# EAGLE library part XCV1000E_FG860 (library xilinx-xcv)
xcv1000e_fg860_1532 edit this description Auto generated by make-symbol-device-package-bsdl.ulp Rev. 26 Source: xcv1000e_fg860_1532.bsd
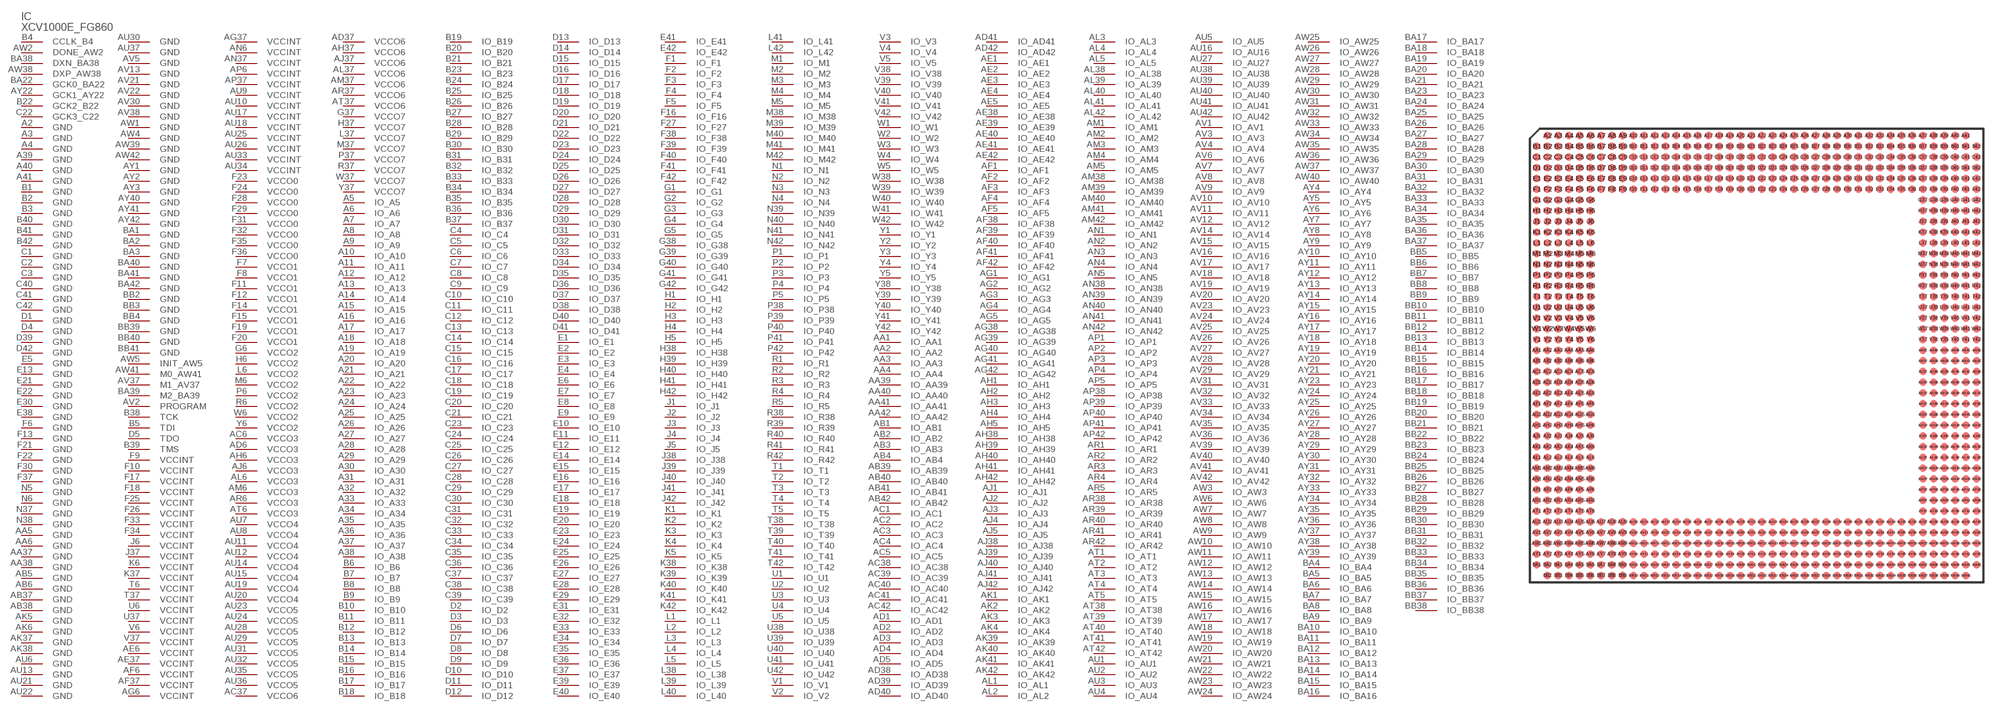
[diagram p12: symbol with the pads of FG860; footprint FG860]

Designator prefix IC

## XCV1000E_FG860 (OC_FARNELL: unknown; OC_NEWARK: unknown)  [FG860]
A2  GND  pwr
A3  GND  pwr
A4  GND  pwr
A5  IO_A5
A6  IO_A6
A7  IO_A7
A8  IO_A8
A9  IO_A9
A10  IO_A10
A11  IO_A11
A12  IO_A12
A13  IO_A13
A14  IO_A14
A15  IO_A15
A16  IO_A16
A17  IO_A17
A18  IO_A18
A19  IO_A19
A20  IO_A20
A21  IO_A21
A22  IO_A22
A23  IO_A23
A24  IO_A24
A25  IO_A25
A26  IO_A26
A27  IO_A27
A28  IO_A28
A29  IO_A29
A30  IO_A30
A31  IO_A31
A32  IO_A32
A33  IO_A33
A34  IO_A34
A35  IO_A35
A36  IO_A36
A37  IO_A37
A38  IO_A38
A39  GND  pwr
A40  GND  pwr
A41  GND  pwr
AA1  IO_AA1
AA2  IO_AA2
AA3  IO_AA3
AA4  IO_AA4
AA5  GND  pwr
AA6  GND  pwr
AA37  GND  pwr
AA38  GND  pwr
AA39  IO_AA39
AA40  IO_AA40
AA41  IO_AA41
AA42  IO_AA42
AB1  IO_AB1
AB2  IO_AB2
AB3  IO_AB3
AB4  IO_AB4
AB5  GND  pwr
AB6  GND  pwr
AB37  GND  pwr
AB38  GND  pwr
AB39  IO_AB39
AB40  IO_AB40
AB41  IO_AB41
AB42  IO_AB42
AC1  IO_AC1
AC2  IO_AC2
AC3  IO_AC3
AC4  IO_AC4
AC5  IO_AC5
AC6  VCCO3  pwr
AC37  VCCO6  pwr
AC38  IO_AC38
AC39  IO_AC39
AC40  IO_AC40
AC41  IO_AC41
AC42  IO_AC42
AD1  IO_AD1
AD2  IO_AD2
AD3  IO_AD3
AD4  IO_AD4
AD5  IO_AD5
AD6  VCCO3  pwr
AD37  VCCO6  pwr
AD38  IO_AD38
AD39  IO_AD39
AD40  IO_AD40
AD41  IO_AD41
AD42  IO_AD42
AE1  IO_AE1
AE2  IO_AE2
AE3  IO_AE3
AE4  IO_AE4
AE5  IO_AE5
AE6  VCCINT  pwr
AE37  VCCINT  pwr
AE38  IO_AE38
AE39  IO_AE39
AE40  IO_AE40
AE41  IO_AE41
AE42  IO_AE42
AF1  IO_AF1
AF2  IO_AF2
AF3  IO_AF3
AF4  IO_AF4
AF5  IO_AF5
AF6  VCCINT  pwr
AF37  VCCINT  pwr
AF38  IO_AF38
AF39  IO_AF39
AF40  IO_AF40
AF41  IO_AF41
AF42  IO_AF42
AG1  IO_AG1
AG2  IO_AG2
AG3  IO_AG3
AG4  IO_AG4
AG5  IO_AG5
AG6  VCCINT  pwr
AG37  VCCINT  pwr
AG38  IO_AG38
AG39  IO_AG39
AG40  IO_AG40
AG41  IO_AG41
AG42  IO_AG42
AH1  IO_AH1
AH2  IO_AH2
AH3  IO_AH3
AH4  IO_AH4
AH5  IO_AH5
AH6  VCCO3  pwr
AH37  VCCO6  pwr
AH38  IO_AH38
AH39  IO_AH39
AH40  IO_AH40
AH41  IO_AH41
AH42  IO_AH42
AJ1  IO_AJ1
AJ2  IO_AJ2
AJ3  IO_AJ3
AJ4  IO_AJ4
AJ5  IO_AJ5
AJ6  VCCO3  pwr
AJ37  VCCO6  pwr
AJ38  IO_AJ38
AJ39  IO_AJ39
AJ40  IO_AJ40
AJ41  IO_AJ41
AJ42  IO_AJ42
AK1  IO_AK1
AK2  IO_AK2
AK3  IO_AK3
AK4  IO_AK4
AK5  GND  pwr
AK6  GND  pwr
AK37  GND  pwr
AK38  GND  pwr
AK39  IO_AK39
AK40  IO_AK40
AK41  IO_AK41
AK42  IO_AK42
AL1  IO_AL1
AL2  IO_AL2
AL3  IO_AL3
AL4  IO_AL4
AL5  IO_AL5
AL6  VCCO3  pwr
AL37  VCCO6  pwr
AL38  IO_AL38
AL39  IO_AL39
AL40  IO_AL40
AL41  IO_AL41
AL42  IO_AL42
AM1  IO_AM1
AM2  IO_AM2
AM3  IO_AM3
AM4  IO_AM4
AM5  IO_AM5
AM6  VCCO3  pwr
AM37  VCCO6  pwr
AM38  IO_AM38
AM39  IO_AM39
AM40  IO_AM40
AM41  IO_AM41
AM42  IO_AM42
AN1  IO_AN1
AN2  IO_AN2
AN3  IO_AN3
AN4  IO_AN4
AN5  IO_AN5
AN6  VCCINT  pwr
AN37  VCCINT  pwr
AN38  IO_AN38
AN39  IO_AN39
AN40  IO_AN40
AN41  IO_AN41
AN42  IO_AN42
AP1  IO_AP1
AP2  IO_AP2
AP3  IO_AP3
AP4  IO_AP4
AP5  IO_AP5
AP6  VCCINT  pwr
AP37  VCCINT  pwr
AP38  IO_AP38
AP39  IO_AP39
AP40  IO_AP40
AP41  IO_AP41
AP42  IO_AP42
AR1  IO_AR1
AR2  IO_AR2
AR3  IO_AR3
AR4  IO_AR4
AR5  IO_AR5
AR6  VCCO3  pwr
AR37  VCCO6  pwr
AR38  IO_AR38
AR39  IO_AR39
AR40  IO_AR40
AR41  IO_AR41
AR42  IO_AR42
AT1  IO_AT1
AT2  IO_AT2
AT3  IO_AT3
AT4  IO_AT4
AT5  IO_AT5
AT6  VCCO3  pwr
AT37  VCCO6  pwr
AT38  IO_AT38
AT39  IO_AT39
AT40  IO_AT40
AT41  IO_AT41
AT42  IO_AT42
AU1  IO_AU1
AU2  IO_AU2
AU3  IO_AU3
AU4  IO_AU4
AU5  IO_AU5
AU6  GND  pwr
AU7  VCCO4  pwr
AU8  VCCO4  pwr
AU9  VCCINT  pwr
AU10  VCCINT  pwr
AU11  VCCO4  pwr
AU12  VCCO4  pwr
AU13  GND  pwr
AU14  VCCO4  pwr
AU15  VCCO4  pwr
AU16  IO_AU16
AU17  VCCINT  pwr
AU18  VCCINT  pwr
AU19  VCCO4  pwr
AU20  VCCO4  pwr
AU21  GND  pwr
AU22  GND  pwr
AU23  VCCO5  pwr
AU24  VCCO5  pwr
AU25  VCCINT  pwr
AU26  VCCINT  pwr
AU27  IO_AU27
AU28  VCCO5  pwr
AU29  VCCO5  pwr
AU30  GND  pwr
AU31  VCCO5  pwr
AU32  VCCO5  pwr
AU33  VCCINT  pwr
AU34  VCCINT  pwr
AU35  VCCO5  pwr
AU36  VCCO5  pwr
AU37  GND  pwr
AU38  IO_AU38
AU39  IO_AU39
AU40  IO_AU40
AU41  IO_AU41
AU42  IO_AU42
AV1  IO_AV1
AV2  PROGRAM  in
AV3  IO_AV3
AV4  IO_AV4
AV5  GND  pwr
AV6  IO_AV6
AV7  IO_AV7
AV8  IO_AV8
AV9  IO_AV9
AV10  IO_AV10
AV11  IO_AV11
AV12  IO_AV12
AV13  GND  pwr
AV14  IO_AV14
AV15  IO_AV15
AV16  IO_AV16
AV17  IO_AV17
AV18  IO_AV18
AV19  IO_AV19
AV20  IO_AV20
AV21  GND  pwr
AV22  GND  pwr
AV23  IO_AV23
AV24  IO_AV24
AV25  IO_AV25
AV26  IO_AV26
AV27  IO_AV27
AV28  IO_AV28
AV29  IO_AV29
AV30  GND  pwr
AV31  IO_AV31
AV32  IO_AV32
AV33  IO_AV33
AV34  IO_AV34
AV35  IO_AV35
AV36  IO_AV36
AV37  M1_AV37  in
AV38  GND  pwr
AV39  IO_AV39
AV40  IO_AV40
AV41  IO_AV41
AV42  IO_AV42
AW1  GND  pwr
AW2  DONE_AW2
AW3  IO_AW3
AW4  GND  pwr
AW5  INIT_AW5
AW6  IO_AW6
AW7  IO_AW7
AW8  IO_AW8
AW9  IO_AW9
AW10  IO_AW10
AW11  IO_AW11
AW12  IO_AW12
AW13  IO_AW13
AW14  IO_AW14
AW15  IO_AW15
AW16  IO_AW16
AW17  IO_AW17
AW18  IO_AW18
AW19  IO_AW19
AW20  IO_AW20
AW21  IO_AW21
AW22  IO_AW22
AW23  IO_AW23
AW24  IO_AW24
AW25  IO_AW25
AW26  IO_AW26
AW27  IO_AW27
AW28  IO_AW28
AW29  IO_AW29
AW30  IO_AW30
AW31  IO_AW31
AW32  IO_AW32
AW33  IO_AW33
AW34  IO_AW34
AW35  IO_AW35
AW36  IO_AW36
AW37  IO_AW37
AW38  DXP_AW38  pas
AW39  GND  pwr
AW40  IO_AW40
AW41  M0_AW41  in
AW42  GND  pwr
AY1  GND  pwr
AY2  GND  pwr
AY3  GND  pwr
AY4  IO_AY4
AY5  IO_AY5
AY6  IO_AY6
AY7  IO_AY7
AY8  IO_AY8
AY9  IO_AY9
AY10  IO_AY10
AY11  IO_AY11
AY12  IO_AY12
AY13  IO_AY13
AY14  IO_AY14
AY15  IO_AY15
AY16  IO_AY16
AY17  IO_AY17
AY18  IO_AY18
AY19  IO_AY19
AY20  IO_AY20
AY21  IO_AY21
AY22  GCK1_AY22  in
AY23  IO_AY23
AY24  IO_AY24
AY25  IO_AY25
AY26  IO_AY26
AY27  IO_AY27
AY28  IO_AY28
AY29  IO_AY29
AY30  IO_AY30
AY31  IO_AY31
AY32  IO_AY32
AY33  IO_AY33
AY34  IO_AY34
AY35  IO_AY35
AY36  IO_AY36
AY37  IO_AY37
AY38  IO_AY38
AY39  IO_AY39
AY40  GND  pwr
AY41  GND  pwr
AY42  GND  pwr
B1  GND  pwr
B2  GND  pwr
B3  GND  pwr
B4  CCLK_B4
B5  TDI  in
B6  IO_B6
B7  IO_B7
B8  IO_B8
B9  IO_B9
B10  IO_B10
B11  IO_B11
B12  IO_B12
B13  IO_B13
B14  IO_B14
B15  IO_B15
B16  IO_B16
B17  IO_B17
B18  IO_B18
B19  IO_B19
B20  IO_B20
B21  IO_B21
B22  GCK2_B22  in
B23  IO_B23
B24  IO_B24
B25  IO_B25
B26  IO_B26
B27  IO_B27
B28  IO_B28
B29  IO_B29
B30  IO_B30
B31  IO_B31
B32  IO_B32
B33  IO_B33
B34  IO_B34
B35  IO_B35
B36  IO_B36
B37  IO_B37
B38  TCK  in
B39  TMS  in
B40  GND  pwr
B41  GND  pwr
B42  GND  pwr
BA1  GND  pwr
BA2  GND  pwr
BA3  GND  pwr
BA4  IO_BA4
BA5  IO_BA5
BA6  IO_BA6
BA7  IO_BA7
BA8  IO_BA8
BA9  IO_BA9
BA10  IO_BA10
BA11  IO_BA11
BA12  IO_BA12
BA13  IO_BA13
BA14  IO_BA14
BA15  IO_BA15
BA16  IO_BA16
BA17  IO_BA17
BA18  IO_BA18
BA19  IO_BA19
BA20  IO_BA20
BA21  IO_BA21
BA22  GCK0_BA22  in
BA23  IO_BA23
BA24  IO_BA24
BA25  IO_BA25
BA26  IO_BA26
BA27  IO_BA27
BA28  IO_BA28
BA29  IO_BA29
BA30  IO_BA30
BA31  IO_BA31
BA32  IO_BA32
BA33  IO_BA33
BA34  IO_BA34
BA35  IO_BA35
BA36  IO_BA36
BA37  IO_BA37
BA38  DXN_BA38  pas
BA39  M2_BA39  in
BA40  GND  pwr
BA41  GND  pwr
BA42  GND  pwr
BB2  GND  pwr
BB3  GND  pwr
BB4  GND  pwr
BB5  IO_BB5
BB6  IO_BB6
BB7  IO_BB7
BB8  IO_BB8
BB9  IO_BB9
BB10  IO_BB10
BB11  IO_BB11
BB12  IO_BB12
BB13  IO_BB13
BB14  IO_BB14
BB15  IO_BB15
BB16  IO_BB16
BB17  IO_BB17
BB18  IO_BB18
BB19  IO_BB19
BB20  IO_BB20
BB21  IO_BB21
BB22  IO_BB22
BB23  IO_BB23
BB24  IO_BB24
BB25  IO_BB25
BB26  IO_BB26
BB27  IO_BB27
BB28  IO_BB28
BB29  IO_BB29
BB30  IO_BB30
BB31  IO_BB31
BB32  IO_BB32
BB33  IO_BB33
BB34  IO_BB34
BB35  IO_BB35
BB36  IO_BB36
BB37  IO_BB37
BB38  IO_BB38
BB39  GND  pwr
BB40  GND  pwr
BB41  GND  pwr
C1  GND  pwr
C2  GND  pwr
C3  GND  pwr
C4  IO_C4
C5  IO_C5
C6  IO_C6
C7  IO_C7
C8  IO_C8
C9  IO_C9
C10  IO_C10
C11  IO_C11
C12  IO_C12
C13  IO_C13
C14  IO_C14
C15  IO_C15
C16  IO_C16
C17  IO_C17
C18  IO_C18
C19  IO_C19
C20  IO_C20
C21  IO_C21
C22  GCK3_C22  in
C23  IO_C23
C24  IO_C24
C25  IO_C25
C26  IO_C26
C27  IO_C27
C28  IO_C28
C29  IO_C29
C30  IO_C30
C31  IO_C31
C32  IO_C32
C33  IO_C33
C34  IO_C34
C35  IO_C35
C36  IO_C36
C37  IO_C37
C38  IO_C38
C39  IO_C39
C40  GND  pwr
C41  GND  pwr
C42  GND  pwr
D1  GND  pwr
D2  IO_D2
D3  IO_D3
D4  GND  pwr
D5  TDO  out
D6  IO_D6
D7  IO_D7
D8  IO_D8
D9  IO_D9
D10  IO_D10
D11  IO_D11
D12  IO_D12
D13  IO_D13
D14  IO_D14
D15  IO_D15
D16  IO_D16
D17  IO_D17
D18  IO_D18
D19  IO_D19
D20  IO_D20
D21  IO_D21
D22  IO_D22
D23  IO_D23
D24  IO_D24
D25  IO_D25
D26  IO_D26
D27  IO_D27
D28  IO_D28
D29  IO_D29
D30  IO_D30
D31  IO_D31
D32  IO_D32
D33  IO_D33
D34  IO_D34
D35  IO_D35
D36  IO_D36
D37  IO_D37
D38  IO_D38
D39  GND  pwr
D40  IO_D40
D41  IO_D41
D42  GND  pwr
E1  IO_E1
E2  IO_E2
E3  IO_E3
E4  IO_E4
E5  GND  pwr
E6  IO_E6
E7  IO_E7
E8  IO_E8
E9  IO_E9
E10  IO_E10
E11  IO_E11
E12  IO_E12
E13  GND  pwr
E14  IO_E14
E15  IO_E15
E16  IO_E16
E17  IO_E17
E18  IO_E18
E19  IO_E19
E20  IO_E20
E21  GND  pwr
E22  GND  pwr
E23  IO_E23
E24  IO_E24
E25  IO_E25
E26  IO_E26
E27  IO_E27
E28  IO_E28
E29  IO_E29
E30  GND  pwr
E31  IO_E31
E32  IO_E32
E33  IO_E33
E34  IO_E34
E35  IO_E35
E36  IO_E36
E37  IO_E37
E38  GND  pwr
E39  IO_E39
E40  IO_E40
E41  IO_E41
E42  IO_E42
F1  IO_F1
F2  IO_F2
F3  IO_F3
F4  IO_F4
F5  IO_F5
F6  GND  pwr
F7  VCCO1  pwr
F8  VCCO1  pwr
F9  VCCINT  pwr
F10  VCCINT  pwr
F11  VCCO1  pwr
F12  VCCO1  pwr
F13  GND  pwr
F14  VCCO1  pwr
F15  VCCO1  pwr
F16  IO_F16
F17  VCCINT  pwr
F18  VCCINT  pwr
F19  VCCO1  pwr
F20  VCCO1  pwr
F21  GND  pwr
F22  GND  pwr
F23  VCCO0  pwr
F24  VCCO0  pwr
F25  VCCINT  pwr
F26  VCCINT  pwr
F27  IO_F27
F28  VCCO0  pwr
F29  VCCO0  pwr
F30  GND  pwr
F31  VCCO0  pwr
F32  VCCO0  pwr
F33  VCCINT  pwr
F34  VCCINT  pwr
F35  VCCO0  pwr
F36  VCCO0  pwr
F37  GND  pwr
F38  IO_F38
F39  IO_F39
F40  IO_F40
F41  IO_F41
F42  IO_F42
G1  IO_G1
G2  IO_G2
G3  IO_G3
G4  IO_G4
G5  IO_G5
G6  VCCO2  pwr
G37  VCCO7  pwr
G38  IO_G38
G39  IO_G39
G40  IO_G40
G41  IO_G41
G42  IO_G42
H1  IO_H1
H2  IO_H2
H3  IO_H3
H4  IO_H4
H5  IO_H5
H6  VCCO2  pwr
H37  VCCO7  pwr
H38  IO_H38
H39  IO_H39
H40  IO_H40
H41  IO_H41
H42  IO_H42
J1  IO_J1
J2  IO_J2
J3  IO_J3
J4  IO_J4
J5  IO_J5
J6  VCCINT  pwr
J37  VCCINT  pwr
J38  IO_J38
J39  IO_J39
J40  IO_J40
J41  IO_J41
J42  IO_J42
K1  IO_K1
K2  IO_K2
K3  IO_K3
K4  IO_K4
K5  IO_K5
K6  VCCINT  pwr
K37  VCCINT  pwr
K38  IO_K38
K39  IO_K39
K40  IO_K40
K41  IO_K41
K42  IO_K42
L1  IO_L1
L2  IO_L2
L3  IO_L3
L4  IO_L4
L5  IO_L5
L6  VCCO2  pwr
L37  VCCO7  pwr
L38  IO_L38
L39  IO_L39
L40  IO_L40
L41  IO_L41
L42  IO_L42
M1  IO_M1
M2  IO_M2
M3  IO_M3
M4  IO_M4
M5  IO_M5
M6  VCCO2  pwr
M37  VCCO7  pwr
M38  IO_M38
M39  IO_M39
M40  IO_M40
M41  IO_M41
M42  IO_M42
N1  IO_N1
N2  IO_N2
N3  IO_N3
N4  IO_N4
N5  GND  pwr
N6  GND  pwr
N37  GND  pwr
N38  GND  pwr
N39  IO_N39
N40  IO_N40
N41  IO_N41
N42  IO_N42
P1  IO_P1
P2  IO_P2
P3  IO_P3
P4  IO_P4
P5  IO_P5
P6  VCCO2  pwr
P37  VCCO7  pwr
P38  IO_P38
P39  IO_P39
P40  IO_P40
P41  IO_P41
P42  IO_P42
R1  IO_R1
R2  IO_R2
R3  IO_R3
R4  IO_R4
R5  IO_R5
R6  VCCO2  pwr
R37  VCCO7  pwr
R38  IO_R38
R39  IO_R39
R40  IO_R40
R41  IO_R41
R42  IO_R42
T1  IO_T1
T2  IO_T2
T3  IO_T3
T4  IO_T4
T5  IO_T5
T6  VCCINT  pwr
T37  VCCINT  pwr
T38  IO_T38
T39  IO_T39
T40  IO_T40
T41  IO_T41
T42  IO_T42
U1  IO_U1
U2  IO_U2
U3  IO_U3
U4  IO_U4
U5  IO_U5
U6  VCCINT  pwr
U37  VCCINT  pwr
U38  IO_U38
U39  IO_U39
U40  IO_U40
U41  IO_U41
U42  IO_U42
V1  IO_V1
V2  IO_V2
V3  IO_V3
V4  IO_V4
V5  IO_V5
V6  VCCINT  pwr
V37  VCCINT  pwr
V38  IO_V38
V39  IO_V39
V40  IO_V40
V41  IO_V41
V42  IO_V42
W1  IO_W1
W2  IO_W2
W3  IO_W3
W4  IO_W4
W5  IO_W5
W6  VCCO2  pwr
W37  VCCO7  pwr
W38  IO_W38
W39  IO_W39
W40  IO_W40
W41  IO_W41
W42  IO_W42
Y1  IO_Y1
Y2  IO_Y2
Y3  IO_Y3
Y4  IO_Y4
Y5  IO_Y5
Y6  VCCO2  pwr
Y37  VCCO7  pwr
Y38  IO_Y38
Y39  IO_Y39
Y40  IO_Y40
Y41  IO_Y41
Y42  IO_Y42

## Footprint FG860 (pad centres in mm)
xcv1000e_fg860_1532 edit this description Auto generated by make-symbol-device-package-bsdl.ulp Rev. 26 Source: xcv1000e_fg860_1532.bsd
smd 0.7 x 0.7: A2 -19.5,20.5; A3 -18.5,20.5; A4 -17.5,20.5; A5 -16.5,20.5; A6 -15.5,20.5; A7 -14.5,20.5; A8 -13.5,20.5; A9 -12.5,20.5; A10 -11.5,20.5; A11 -10.5,20.5; A12 -9.5,20.5; A13 -8.5,20.5; A14 -7.5,20.5; A15 -6.5,20.5; A16 -5.5,20.5; A17 -4.5,20.5; A18 -3.5,20.5; A19 -2.5,20.5; A20 -1.5,20.5; A21 -0.5,20.5; A22 0.5,20.5; A23 1.5,20.5; A24 2.5,20.5; A25 3.5,20.5; A26 4.5,20.5; A27 5.5,20.5; A28 6.5,20.5; A29 7.5,20.5; A30 8.5,20.5; A31 9.5,20.5; A32 10.5,20.5; A33 11.5,20.5; A34 12.5,20.5; A35 13.5,20.5; A36 14.5,20.5; A37 15.5,20.5; A38 16.5,20.5; A39 17.5,20.5; A40 18.5,20.5; A41 19.5,20.5; AA1 -20.5,0.5; AA2 -19.5,0.5; AA3 -18.5,0.5; AA4 -17.5,0.5; AA5 -16.5,0.5; AA6 -15.5,0.5; AA37 15.5,0.5; AA38 16.5,0.5; AA39 17.5,0.5; AA40 18.5,0.5; AA41 19.5,0.5; AA42 20.5,0.5; AB1 -20.5,-0.5; AB2 -19.5,-0.5; AB3 -18.5,-0.5; AB4 -17.5,-0.5; AB5 -16.5,-0.5; AB6 -15.5,-0.5; AB37 15.5,-0.5; AB38 16.5,-0.5; AB39 17.5,-0.5; AB40 18.5,-0.5; AB41 19.5,-0.5; AB42 20.5,-0.5; AC1 -20.5,-1.5; AC2 -19.5,-1.5; AC3 -18.5,-1.5; AC4 -17.5,-1.5; AC5 -16.5,-1.5; AC6 -15.5,-1.5; AC37 15.5,-1.5; AC38 16.5,-1.5; AC39 17.5,-1.5; AC40 18.5,-1.5; AC41 19.5,-1.5; AC42 20.5,-1.5; AD1 -20.5,-2.5; AD2 -19.5,-2.5; AD3 -18.5,-2.5; AD4 -17.5,-2.5; AD5 -16.5,-2.5; AD6 -15.5,-2.5; AD37 15.5,-2.5; AD38 16.5,-2.5; AD39 17.5,-2.5; AD40 18.5,-2.5; AD41 19.5,-2.5; AD42 20.5,-2.5; AE1 -20.5,-3.5; AE2 -19.5,-3.5; AE3 -18.5,-3.5; AE4 -17.5,-3.5; AE5 -16.5,-3.5; AE6 -15.5,-3.5; AE37 15.5,-3.5; AE38 16.5,-3.5; AE39 17.5,-3.5; AE40 18.5,-3.5; AE41 19.5,-3.5; AE42 20.5,-3.5; AF1 -20.5,-4.5; AF2 -19.5,-4.5; AF3 -18.5,-4.5; AF4 -17.5,-4.5; AF5 -16.5,-4.5; AF6 -15.5,-4.5; AF37 15.5,-4.5; AF38 16.5,-4.5; AF39 17.5,-4.5; AF40 18.5,-4.5; AF41 19.5,-4.5; AF42 20.5,-4.5; AG1 -20.5,-5.5; AG2 -19.5,-5.5; AG3 -18.5,-5.5; AG4 -17.5,-5.5; AG5 -16.5,-5.5; AG6 -15.5,-5.5; AG37 15.5,-5.5; AG38 16.5,-5.5; AG39 17.5,-5.5; AG40 18.5,-5.5; AG41 19.5,-5.5; AG42 20.5,-5.5; AH1 -20.5,-6.5; AH2 -19.5,-6.5; AH3 -18.5,-6.5; AH4 -17.5,-6.5; AH5 -16.5,-6.5; AH6 -15.5,-6.5; AH37 15.5,-6.5; AH38 16.5,-6.5; AH39 17.5,-6.5; AH40 18.5,-6.5; AH41 19.5,-6.5; AH42 20.5,-6.5; AJ1 -20.5,-7.5; AJ2 -19.5,-7.5; AJ3 -18.5,-7.5; AJ4 -17.5,-7.5; AJ5 -16.5,-7.5; AJ6 -15.5,-7.5; AJ37 15.5,-7.5; AJ38 16.5,-7.5; AJ39 17.5,-7.5; AJ40 18.5,-7.5; AJ41 19.5,-7.5; AJ42 20.5,-7.5; AK1 -20.5,-8.5; AK2 -19.5,-8.5; AK3 -18.5,-8.5; AK4 -17.5,-8.5; AK5 -16.5,-8.5; AK6 -15.5,-8.5; AK37 15.5,-8.5; AK38 16.5,-8.5; AK39 17.5,-8.5; AK40 18.5,-8.5; AK41 19.5,-8.5; AK42 20.5,-8.5; AL1 -20.5,-9.5; AL2 -19.5,-9.5; AL3 -18.5,-9.5; AL4 -17.5,-9.5; AL5 -16.5,-9.5; AL6 -15.5,-9.5; AL37 15.5,-9.5; AL38 16.5,-9.5; AL39 17.5,-9.5; AL40 18.5,-9.5; AL41 19.5,-9.5; AL42 20.5,-9.5; AM1 -20.5,-10.5; AM2 -19.5,-10.5; AM3 -18.5,-10.5; AM4 -17.5,-10.5; AM5 -16.5,-10.5; AM6 -15.5,-10.5; AM37 15.5,-10.5; AM38 16.5,-10.5; AM39 17.5,-10.5; AM40 18.5,-10.5; AM41 19.5,-10.5; AM42 20.5,-10.5; AN1 -20.5,-11.5; AN2 -19.5,-11.5; AN3 -18.5,-11.5; AN4 -17.5,-11.5; AN5 -16.5,-11.5; AN6 -15.5,-11.5; AN37 15.5,-11.5; AN38 16.5,-11.5; AN39 17.5,-11.5; AN40 18.5,-11.5; AN41 19.5,-11.5; AN42 20.5,-11.5; AP1 -20.5,-12.5; AP2 -19.5,-12.5; AP3 -18.5,-12.5; AP4 -17.5,-12.5; AP5 -16.5,-12.5; AP6 -15.5,-12.5; AP37 15.5,-12.5; AP38 16.5,-12.5; AP39 17.5,-12.5; AP40 18.5,-12.5; AP41 19.5,-12.5; AP42 20.5,-12.5; AR1 -20.5,-13.5; AR2 -19.5,-13.5; AR3 -18.5,-13.5; AR4 -17.5,-13.5; AR5 -16.5,-13.5; AR6 -15.5,-13.5; AR37 15.5,-13.5; AR38 16.5,-13.5; AR39 17.5,-13.5; AR40 18.5,-13.5; AR41 19.5,-13.5; AR42 20.5,-13.5; AT1 -20.5,-14.5; AT2 -19.5,-14.5; AT3 -18.5,-14.5; AT4 -17.5,-14.5; AT5 -16.5,-14.5; AT6 -15.5,-14.5; AT37 15.5,-14.5; AT38 16.5,-14.5; AT39 17.5,-14.5; AT40 18.5,-14.5; AT41 19.5,-14.5; AT42 20.5,-14.5; AU1 -20.5,-15.5; AU2 -19.5,-15.5; AU3 -18.5,-15.5; AU4 -17.5,-15.5; AU5 -16.5,-15.5; AU6 -15.5,-15.5; AU7 -14.5,-15.5; AU8 -13.5,-15.5; AU9 -12.5,-15.5; AU10 -11.5,-15.5; AU11 -10.5,-15.5; AU12 -9.5,-15.5; AU13 -8.5,-15.5; AU14 -7.5,-15.5; AU15 -6.5,-15.5; AU16 -5.5,-15.5; AU17 -4.5,-15.5; AU18 -3.5,-15.5; AU19 -2.5,-15.5; AU20 -1.5,-15.5; AU21 -0.5,-15.5; AU22 0.5,-15.5; AU23 1.5,-15.5; AU24 2.5,-15.5; AU25 3.5,-15.5; AU26 4.5,-15.5; AU27 5.5,-15.5; AU28 6.5,-15.5; AU29 7.5,-15.5; AU30 8.5,-15.5; AU31 9.5,-15.5; AU32 10.5,-15.5; AU33 11.5,-15.5; AU34 12.5,-15.5; AU35 13.5,-15.5; AU36 14.5,-15.5; AU37 15.5,-15.5; AU38 16.5,-15.5; AU39 17.5,-15.5; AU40 18.5,-15.5; AU41 19.5,-15.5; AU42 20.5,-15.5; AV1 -20.5,-16.5; AV2 -19.5,-16.5; AV3 -18.5,-16.5; AV4 -17.5,-16.5; AV5 -16.5,-16.5; AV6 -15.5,-16.5; AV7 -14.5,-16.5; AV8 -13.5,-16.5; AV9 -12.5,-16.5; AV10 -11.5,-16.5; AV11 -10.5,-16.5; AV12 -9.5,-16.5; AV13 -8.5,-16.5; AV14 -7.5,-16.5; AV15 -6.5,-16.5; AV16 -5.5,-16.5; AV17 -4.5,-16.5; AV18 -3.5,-16.5; AV19 -2.5,-16.5; AV20 -1.5,-16.5; AV21 -0.5,-16.5; AV22 0.5,-16.5; AV23 1.5,-16.5; AV24 2.5,-16.5; AV25 3.5,-16.5; AV26 4.5,-16.5; AV27 5.5,-16.5; AV28 6.5,-16.5; AV29 7.5,-16.5; AV30 8.5,-16.5; AV31 9.5,-16.5; AV32 10.5,-16.5; AV33 11.5,-16.5; AV34 12.5,-16.5; AV35 13.5,-16.5; AV36 14.5,-16.5; AV37 15.5,-16.5; AV38 16.5,-16.5; AV39 17.5,-16.5; AV40 18.5,-16.5; AV41 19.5,-16.5; AV42 20.5,-16.5; AW1 -20.5,-17.5; AW2 -19.5,-17.5; AW3 -18.5,-17.5; AW4 -17.5,-17.5; AW5 -16.5,-17.5; AW6 -15.5,-17.5; AW7 -14.5,-17.5; AW8 -13.5,-17.5; AW9 -12.5,-17.5; AW10 -11.5,-17.5; AW11 -10.5,-17.5; AW12 -9.5,-17.5; AW13 -8.5,-17.5; AW14 -7.5,-17.5; AW15 -6.5,-17.5; AW16 -5.5,-17.5; AW17 -4.5,-17.5; AW18 -3.5,-17.5; AW19 -2.5,-17.5; AW20 -1.5,-17.5; AW21 -0.5,-17.5; AW22 0.5,-17.5; AW23 1.5,-17.5; AW24 2.5,-17.5; AW25 3.5,-17.5; AW26 4.5,-17.5; AW27 5.5,-17.5; AW28 6.5,-17.5; AW29 7.5,-17.5; AW30 8.5,-17.5; AW31 9.5,-17.5; AW32 10.5,-17.5; AW33 11.5,-17.5; AW34 12.5,-17.5; AW35 13.5,-17.5; AW36 14.5,-17.5; AW37 15.5,-17.5; AW38 16.5,-17.5; AW39 17.5,-17.5; AW40 18.5,-17.5; AW41 19.5,-17.5; AW42 20.5,-17.5; AY1 -20.5,-18.5; AY2 -19.5,-18.5; AY3 -18.5,-18.5; AY4 -17.5,-18.5; AY5 -16.5,-18.5; AY6 -15.5,-18.5; AY7 -14.5,-18.5; AY8 -13.5,-18.5; AY9 -12.5,-18.5; AY10 -11.5,-18.5; AY11 -10.5,-18.5; AY12 -9.5,-18.5; AY13 -8.5,-18.5; AY14 -7.5,-18.5; AY15 -6.5,-18.5; AY16 -5.5,-18.5; AY17 -4.5,-18.5; AY18 -3.5,-18.5; AY19 -2.5,-18.5; AY20 -1.5,-18.5; AY21 -0.5,-18.5; AY22 0.5,-18.5; AY23 1.5,-18.5; AY24 2.5,-18.5; AY25 3.5,-18.5; AY26 4.5,-18.5; AY27 5.5,-18.5; AY28 6.5,-18.5; AY29 7.5,-18.5; AY30 8.5,-18.5; AY31 9.5,-18.5; AY32 10.5,-18.5; AY33 11.5,-18.5; AY34 12.5,-18.5; AY35 13.5,-18.5; AY36 14.5,-18.5; AY37 15.5,-18.5; AY38 16.5,-18.5; AY39 17.5,-18.5; AY40 18.5,-18.5; AY41 19.5,-18.5; AY42 20.5,-18.5; B1 -20.5,19.5; B2 -19.5,19.5; B3 -18.5,19.5; B4 -17.5,19.5; B5 -16.5,19.5; B6 -15.5,19.5; B7 -14.5,19.5; B8 -13.5,19.5; B9 -12.5,19.5; B10 -11.5,19.5; B11 -10.5,19.5; B12 -9.5,19.5; B13 -8.5,19.5; B14 -7.5,19.5; B15 -6.5,19.5; B16 -5.5,19.5; B17 -4.5,19.5; B18 -3.5,19.5; B19 -2.5,19.5; B20 -1.5,19.5; B21 -0.5,19.5; B22 0.5,19.5; B23 1.5,19.5; B24 2.5,19.5; B25 3.5,19.5; B26 4.5,19.5; B27 5.5,19.5; B28 6.5,19.5; B29 7.5,19.5; B30 8.5,19.5; B31 9.5,19.5; B32 10.5,19.5; B33 11.5,19.5; B34 12.5,19.5; B35 13.5,19.5; B36 14.5,19.5; B37 15.5,19.5; B38 16.5,19.5; B39 17.5,19.5; B40 18.5,19.5; B41 19.5,19.5; B42 20.5,19.5; BA1 -20.5,-19.5; BA2 -19.5,-19.5; BA3 -18.5,-19.5; BA4 -17.5,-19.5; BA5 -16.5,-19.5; BA6 -15.5,-19.5; BA7 -14.5,-19.5; BA8 -13.5,-19.5; BA9 -12.5,-19.5; BA10 -11.5,-19.5; BA11 -10.5,-19.5; BA12 -9.5,-19.5; BA13 -8.5,-19.5; BA14 -7.5,-19.5; BA15 -6.5,-19.5; BA16 -5.5,-19.5; BA17 -4.5,-19.5; BA18 -3.5,-19.5; BA19 -2.5,-19.5; BA20 -1.5,-19.5; BA21 -0.5,-19.5; BA22 0.5,-19.5; BA23 1.5,-19.5; BA24 2.5,-19.5; BA25 3.5,-19.5; BA26 4.5,-19.5; BA27 5.5,-19.5; BA28 6.5,-19.5; BA29 7.5,-19.5; BA30 8.5,-19.5; BA31 9.5,-19.5; BA32 10.5,-19.5; BA33 11.5,-19.5; BA34 12.5,-19.5; BA35 13.5,-19.5; BA36 14.5,-19.5; BA37 15.5,-19.5; BA38 16.5,-19.5; BA39 17.5,-19.5; BA40 18.5,-19.5; BA41 19.5,-19.5; BA42 20.5,-19.5; BB2 -19.5,-20.5; BB3 -18.5,-20.5; BB4 -17.5,-20.5; BB5 -16.5,-20.5; BB6 -15.5,-20.5; BB7 -14.5,-20.5; BB8 -13.5,-20.5; BB9 -12.5,-20.5; BB10 -11.5,-20.5; BB11 -10.5,-20.5; BB12 -9.5,-20.5; BB13 -8.5,-20.5; BB14 -7.5,-20.5; BB15 -6.5,-20.5; BB16 -5.5,-20.5; BB17 -4.5,-20.5; BB18 -3.5,-20.5; BB19 -2.5,-20.5; BB20 -1.5,-20.5; BB21 -0.5,-20.5; BB22 0.5,-20.5; BB23 1.5,-20.5; BB24 2.5,-20.5; BB25 3.5,-20.5; BB26 4.5,-20.5; BB27 5.5,-20.5; BB28 6.5,-20.5; BB29 7.5,-20.5; BB30 8.5,-20.5; BB31 9.5,-20.5; BB32 10.5,-20.5; BB33 11.5,-20.5; BB34 12.5,-20.5; BB35 13.5,-20.5; BB36 14.5,-20.5; BB37 15.5,-20.5; BB38 16.5,-20.5; BB39 17.5,-20.5; BB40 18.5,-20.5; BB41 19.5,-20.5; C1 -20.5,18.5; C2 -19.5,18.5; C3 -18.5,18.5; C4 -17.5,18.5; C5 -16.5,18.5; C6 -15.5,18.5; C7 -14.5,18.5; C8 -13.5,18.5; C9 -12.5,18.5; C10 -11.5,18.5; C11 -10.5,18.5; C12 -9.5,18.5; C13 -8.5,18.5; C14 -7.5,18.5; C15 -6.5,18.5; C16 -5.5,18.5; C17 -4.5,18.5; C18 -3.5,18.5; C19 -2.5,18.5; C20 -1.5,18.5; C21 -0.5,18.5; C22 0.5,18.5; C23 1.5,18.5; C24 2.5,18.5; C25 3.5,18.5; C26 4.5,18.5; C27 5.5,18.5; C28 6.5,18.5; C29 7.5,18.5; C30 8.5,18.5; C31 9.5,18.5; C32 10.5,18.5; C33 11.5,18.5; C34 12.5,18.5; C35 13.5,18.5; C36 14.5,18.5; C37 15.5,18.5; C38 16.5,18.5; C39 17.5,18.5; C40 18.5,18.5; C41 19.5,18.5; C42 20.5,18.5; D1 -20.5,17.5; D2 -19.5,17.5; D3 -18.5,17.5; D4 -17.5,17.5; D5 -16.5,17.5; D6 -15.5,17.5; D7 -14.5,17.5; D8 -13.5,17.5; D9 -12.5,17.5; D10 -11.5,17.5; D11 -10.5,17.5; D12 -9.5,17.5; D13 -8.5,17.5; D14 -7.5,17.5; D15 -6.5,17.5; D16 -5.5,17.5; D17 -4.5,17.5; D18 -3.5,17.5; D19 -2.5,17.5; D20 -1.5,17.5; D21 -0.5,17.5; D22 0.5,17.5; D23 1.5,17.5; D24 2.5,17.5; D25 3.5,17.5; D26 4.5,17.5; D27 5.5,17.5; D28 6.5,17.5; D29 7.5,17.5; D30 8.5,17.5; D31 9.5,17.5; D32 10.5,17.5; D33 11.5,17.5; D34 12.5,17.5; D35 13.5,17.5; D36 14.5,17.5; D37 15.5,17.5; D38 16.5,17.5; D39 17.5,17.5; D40 18.5,17.5; D41 19.5,17.5; D42 20.5,17.5; E1 -20.5,16.5; E2 -19.5,16.5; E3 -18.5,16.5; E4 -17.5,16.5; E5 -16.5,16.5; E6 -15.5,16.5; E7 -14.5,16.5; E8 -13.5,16.5; E9 -12.5,16.5; E10 -11.5,16.5; E11 -10.5,16.5; E12 -9.5,16.5; E13 -8.5,16.5; E14 -7.5,16.5; E15 -6.5,16.5; E16 -5.5,16.5; E17 -4.5,16.5; E18 -3.5,16.5; E19 -2.5,16.5; E20 -1.5,16.5; E21 -0.5,16.5; E22 0.5,16.5; E23 1.5,16.5; E24 2.5,16.5; E25 3.5,16.5; E26 4.5,16.5; E27 5.5,16.5; E28 6.5,16.5; E29 7.5,16.5; E30 8.5,16.5; E31 9.5,16.5; E32 10.5,16.5; E33 11.5,16.5; E34 12.5,16.5; E35 13.5,16.5; E36 14.5,16.5; E37 15.5,16.5; E38 16.5,16.5; E39 17.5,16.5; E40 18.5,16.5; E41 19.5,16.5; E42 20.5,16.5; F1 -20.5,15.5; F2 -19.5,15.5; F3 -18.5,15.5; F4 -17.5,15.5; F5 -16.5,15.5; F6 -15.5,15.5; F7 -14.5,15.5; F8 -13.5,15.5; F9 -12.5,15.5; F10 -11.5,15.5; F11 -10.5,15.5; F12 -9.5,15.5; F13 -8.5,15.5; F14 -7.5,15.5; F15 -6.5,15.5; F16 -5.5,15.5; F17 -4.5,15.5; F18 -3.5,15.5; F19 -2.5,15.5; F20 -1.5,15.5; F21 -0.5,15.5; F22 0.5,15.5; F23 1.5,15.5; F24 2.5,15.5; F25 3.5,15.5; F26 4.5,15.5; F27 5.5,15.5; F28 6.5,15.5; F29 7.5,15.5; F30 8.5,15.5; F31 9.5,15.5; F32 10.5,15.5; F33 11.5,15.5; F34 12.5,15.5; F35 13.5,15.5; F36 14.5,15.5; F37 15.5,15.5; F38 16.5,15.5; F39 17.5,15.5; F40 18.5,15.5; F41 19.5,15.5; F42 20.5,15.5; G1 -20.5,14.5; G2 -19.5,14.5; G3 -18.5,14.5; G4 -17.5,14.5; G5 -16.5,14.5; G6 -15.5,14.5; G37 15.5,14.5; G38 16.5,14.5; G39 17.5,14.5; G40 18.5,14.5; G41 19.5,14.5; G42 20.5,14.5; H1 -20.5,13.5; H2 -19.5,13.5; H3 -18.5,13.5; H4 -17.5,13.5; H5 -16.5,13.5; H6 -15.5,13.5; H37 15.5,13.5; H38 16.5,13.5; H39 17.5,13.5; H40 18.5,13.5; H41 19.5,13.5; H42 20.5,13.5; J1 -20.5,12.5; J2 -19.5,12.5; J3 -18.5,12.5; J4 -17.5,12.5; J5 -16.5,12.5; J6 -15.5,12.5; J37 15.5,12.5; J38 16.5,12.5; J39 17.5,12.5; J40 18.5,12.5; J41 19.5,12.5; J42 20.5,12.5; K1 -20.5,11.5; K2 -19.5,11.5; K3 -18.5,11.5; K4 -17.5,11.5; K5 -16.5,11.5; K6 -15.5,11.5; K37 15.5,11.5; K38 16.5,11.5; K39 17.5,11.5; K40 18.5,11.5; K41 19.5,11.5; K42 20.5,11.5; L1 -20.5,10.5; L2 -19.5,10.5; L3 -18.5,10.5; L4 -17.5,10.5; L5 -16.5,10.5; L6 -15.5,10.5; L37 15.5,10.5; L38 16.5,10.5; L39 17.5,10.5; L40 18.5,10.5; L41 19.5,10.5; L42 20.5,10.5; M1 -20.5,9.5; M2 -19.5,9.5; M3 -18.5,9.5; M4 -17.5,9.5; M5 -16.5,9.5; M6 -15.5,9.5; M37 15.5,9.5; M38 16.5,9.5; M39 17.5,9.5; M40 18.5,9.5; M41 19.5,9.5; M42 20.5,9.5; N1 -20.5,8.5; N2 -19.5,8.5; N3 -18.5,8.5; N4 -17.5,8.5; N5 -16.5,8.5; N6 -15.5,8.5; N37 15.5,8.5; N38 16.5,8.5; N39 17.5,8.5; N40 18.5,8.5; N41 19.5,8.5; N42 20.5,8.5; P1 -20.5,7.5; P2 -19.5,7.5; P3 -18.5,7.5; P4 -17.5,7.5; P5 -16.5,7.5; P6 -15.5,7.5; P37 15.5,7.5; P38 16.5,7.5; P39 17.5,7.5; P40 18.5,7.5; P41 19.5,7.5; P42 20.5,7.5; R1 -20.5,6.5; R2 -19.5,6.5; R3 -18.5,6.5; R4 -17.5,6.5; R5 -16.5,6.5; R6 -15.5,6.5; R37 15.5,6.5; R38 16.5,6.5; R39 17.5,6.5; R40 18.5,6.5; R41 19.5,6.5; R42 20.5,6.5; T1 -20.5,5.5; T2 -19.5,5.5; T3 -18.5,5.5; T4 -17.5,5.5; T5 -16.5,5.5; T6 -15.5,5.5; T37 15.5,5.5; T38 16.5,5.5; T39 17.5,5.5; T40 18.5,5.5; T41 19.5,5.5; T42 20.5,5.5; U1 -20.5,4.5; U2 -19.5,4.5; U3 -18.5,4.5; U4 -17.5,4.5; U5 -16.5,4.5; U6 -15.5,4.5; U37 15.5,4.5; U38 16.5,4.5; U39 17.5,4.5; U40 18.5,4.5; U41 19.5,4.5; U42 20.5,4.5; V1 -20.5,3.5; V2 -19.5,3.5; V3 -18.5,3.5; V4 -17.5,3.5; V5 -16.5,3.5; V6 -15.5,3.5; V37 15.5,3.5; V38 16.5,3.5; V39 17.5,3.5; V40 18.5,3.5; V41 19.5,3.5; V42 20.5,3.5; W1 -20.5,2.5; W2 -19.5,2.5; W3 -18.5,2.5; W4 -17.5,2.5; W5 -16.5,2.5; W6 -15.5,2.5; W37 15.5,2.5; W38 16.5,2.5; W39 17.5,2.5; W40 18.5,2.5; W41 19.5,2.5; W42 20.5,2.5; Y1 -20.5,1.5; Y2 -19.5,1.5; Y3 -18.5,1.5; Y4 -17.5,1.5; Y5 -16.5,1.5; Y6 -15.5,1.5; Y37 15.5,1.5; Y38 16.5,1.5; Y39 17.5,1.5; Y40 18.5,1.5; Y41 19.5,1.5; Y42 20.5,1.5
